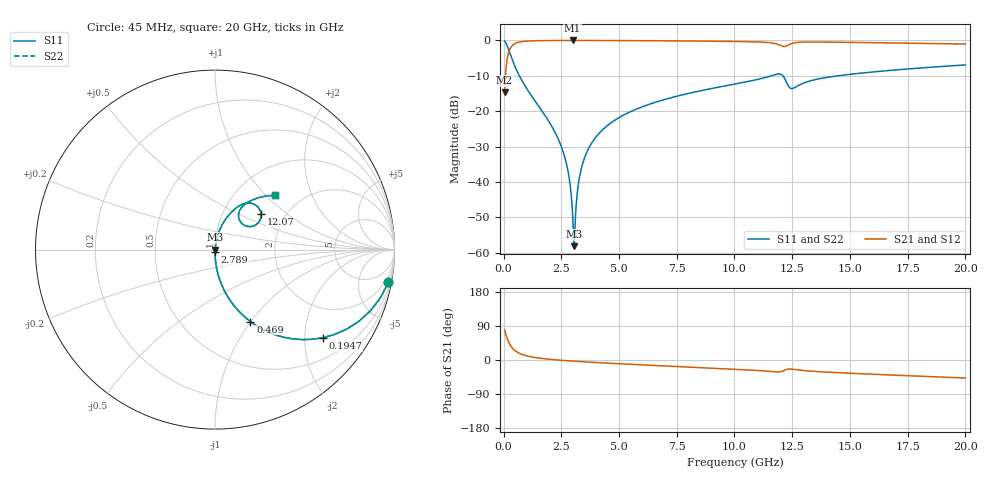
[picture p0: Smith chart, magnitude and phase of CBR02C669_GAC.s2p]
! S-parameter model data by Modelithics Inc.  support@modelithics.com 813-866-6335  Tampa FL USA
! S-Parameter data specifications:
! Substrate: 20-mil Rogers 4350B, substrate thickness, H=0.508mm, Dielectric constant, Er=3.75
! PCB Mounting Pad Footprint: Pad width, PadW=0.32mm , Pad length, PadL=0.37mm , Pad gap, PadG (edge-to-edge)=0.19mm , Reference planes=0.93mm apart
#  GHz  S  MA  R 50
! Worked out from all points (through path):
!   801 points, 45 MHz to 20 GHz, reference 50 ohm
!   highest |S21| = -0.01 dB at 2.988 GHz (marker M1); lowest = -14.7 dB at 45 MHz (marker M2)
!   group delay of S21, straight-line fit = 8.46 ps
!   lowest |S11| = -58.1 dB at 3.063 GHz (marker M3), VSWR 1.00, Z = 50.1 + j0.0429 ohm
!   |S11| at or under -10 dB: 684.5 MHz to 11.59 GHz (10.9 GHz wide, 178 % of centre); 12.1 GHz to 14.47 GHz (2.375 GHz wide, 17.9 % of centre)
!   |S22| runs from -58.1 to -0.1 dB; largest |S21 - S12| = 0
!   S11 on the Smith chart (normalised r, x): 45 MHz: 1, -11; 194.7 MHz: 0.99, -2.45; 469 MHz: 0.99, -1.00; 2.789 GHz: 1.00, -0.03; 12.07 GHz: 1.51, +0.67; 20 GHz: 1.49, +1.13
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0.045  0.9829 -10.7  0.1841 79.3  0.1841 79.3  0.9829 -10.7
0.194662  0.7756 -39.3  0.6307 50.7  0.6307 50.7  0.7756 -39.3
0.469044  0.4472 -63.8  0.8937 26.1  0.8937 26.1  0.4472 -63.8
0.967919  0.2179 -78.2  0.9751 11.6  0.9751 11.6  0.2179 -78.2
2.24005  0.04956 -88.3  0.9977 0.5  0.9977 0.5  0.04956 -88.3
2.564319  0.02769 -88.8  0.9985 -1.1  0.9985 -1.1  0.02769 -88.8
2.788813  0.01437 -87.6  0.9987 -2.1  0.9987 -2.1  0.01437 -87.6
2.888587  0.008844 -85.2  0.9988 -2.5  0.9988 -2.5  0.008844 -85.2
2.988363  0.003594 -74.5  0.9988 -2.9  0.9988 -2.9  0.003594 -74.5
3.063194  0.001244 20.1  0.9988 -3.2  0.9988 -3.2  0.001244 20.1
3.138025  0.004455 71.5  0.9988 -3.5  0.9988 -3.5  0.004455 71.5
3.262744  0.01053 79.7  0.9987 -4.0  0.9987 -4.0  0.01053 79.7
3.387462  0.01646 81.4  0.9986 -4.5  0.9986 -4.5  0.01646 81.4
3.786563  0.03428 82.1  0.9981 -5.9  0.9981 -5.9  0.03428 82.1
4.410156  0.05947 80.8  0.9969 -8.0  0.9969 -8.0  0.05947 80.8
6.704981  0.1381 74.5  0.9888 -14.9  0.9888 -14.9  0.1381 74.5
10.0225  0.2424 64.9  0.9669 -24.4  0.9669 -24.4  0.2424 64.9
12.06789  0.3237 37.6  0.8299 -29.9  0.8299 -29.9  0.3237 37.6
12.46699  0.209 43.8  0.9022 -24.1  0.9022 -24.1  0.209 43.8
13.36496  0.2729 57.8  0.95 -29.7  0.95 -29.7  0.2729 57.8
16.68248  0.376 50.1  0.9231 -39.4  0.9231 -39.4  0.376 50.1
20  0.4506 42.1  0.8896 -47.6  0.8896 -47.6  0.4506 42.1
